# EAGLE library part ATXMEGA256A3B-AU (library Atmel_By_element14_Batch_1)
8/16-bit XMEGA A3 Microcontroller
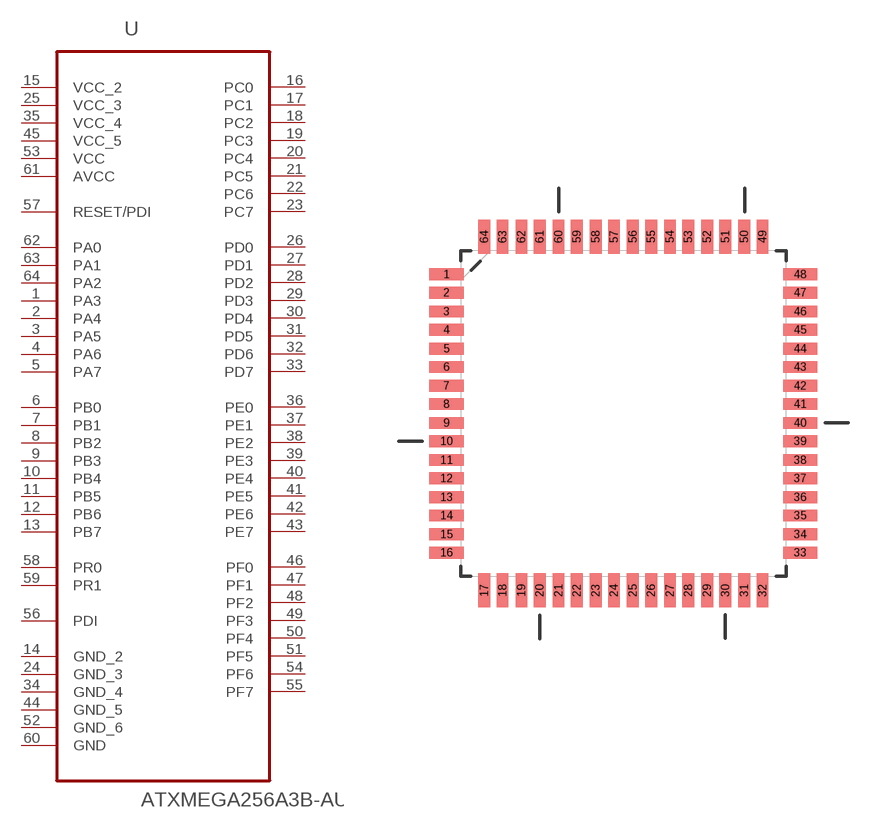
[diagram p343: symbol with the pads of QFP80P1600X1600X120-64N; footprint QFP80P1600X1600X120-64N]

Designator prefix U

## ATXMEGA256A3B-AU (DESCRIPTION: 8/16-bit XMEGA A3 Microcontroller; MPN: ATXMEGA256A3B-AU; OC_FARNELL: 1841632; OC_NEWARK: -; PACKAGE: TQFP-64; SUPPLIER: Atmel Corporation)  [QFP80P1600X1600X120-64N]
1  PA3
2  PA4
3  PA5
4  PA6
5  PA7
6  PB0
7  PB1
8  PB2
9  PB3
10  PB4
11  PB5
12  PB6
13  PB7
14  GND_2  pas
15  VCC_2  pwr
16  PC0
17  PC1
18  PC2
19  PC3
20  PC4
21  PC5
22  PC6
23  PC7
24  GND_3  pas
25  VCC_3  pwr
26  PD0
27  PD1
28  PD2
29  PD3
30  PD4
31  PD5
32  PD6
33  PD7
34  GND_4  pas
35  VCC_4  pwr
36  PE0
37  PE1
38  PE2
39  PE3
40  PE4
41  PE5
42  PE6
43  PE7
44  GND_5  pas
45  VCC_5  pwr
46  PF0
47  PF1
48  PF2
49  PF3
50  PF4
51  PF5
52  GND_6  pas
53  VCC  pwr
54  PF6
55  PF7
56  PDI  pas
57  RESET/PDI  in
58  PR0
59  PR1
60  GND  pas
61  AVCC  pwr
62  PA0
63  PA1
64  PA2

## Footprint QFP80P1600X1600X120-64N (pad centres in mm)
smd 1.473 x 0.508: 1 -7.62,5.994; 2 -7.62,5.207; 3 -7.62,4.394; 4 -7.62,3.607; 5 -7.62,2.794; 6 -7.62,2.007; 7 -7.62,1.194; 8 -7.62,0.406; 9 -7.62,-0.406; 10 -7.62,-1.194; 11 -7.62,-2.007; 12 -7.62,-2.794; 13 -7.62,-3.607; 14 -7.62,-4.394; 15 -7.62,-5.207; 16 -7.62,-5.994; 33 7.62,-5.994; 34 7.62,-5.207; 35 7.62,-4.394; 36 7.62,-3.607; 37 7.62,-2.794; 38 7.62,-2.007; 39 7.62,-1.194; 40 7.62,-0.406; 41 7.62,0.406; 42 7.62,1.194; 43 7.62,2.007; 44 7.62,2.794; 45 7.62,3.607; 46 7.62,4.394; 47 7.62,5.207; 48 7.62,5.994
smd 0.508 x 1.473: 17 -5.994,-7.62; 18 -5.207,-7.62; 19 -4.394,-7.62; 20 -3.607,-7.62; 21 -2.794,-7.62; 22 -2.007,-7.62; 23 -1.194,-7.62; 24 -0.406,-7.62; 25 0.406,-7.62; 26 1.194,-7.62; 27 2.007,-7.62; 28 2.794,-7.62; 29 3.607,-7.62; 30 4.394,-7.62; 31 5.207,-7.62; 32 5.994,-7.62; 49 5.994,7.62; 50 5.207,7.62; 51 4.394,7.62; 52 3.607,7.62; 53 2.794,7.62; 54 2.007,7.62; 55 1.194,7.62; 56 0.406,7.62; 57 -0.406,7.62; 58 -1.194,7.62; 59 -2.007,7.62; 60 -2.794,7.62; 61 -3.607,7.62; 62 -4.394,7.62; 63 -5.207,7.62; 64 -5.994,7.62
